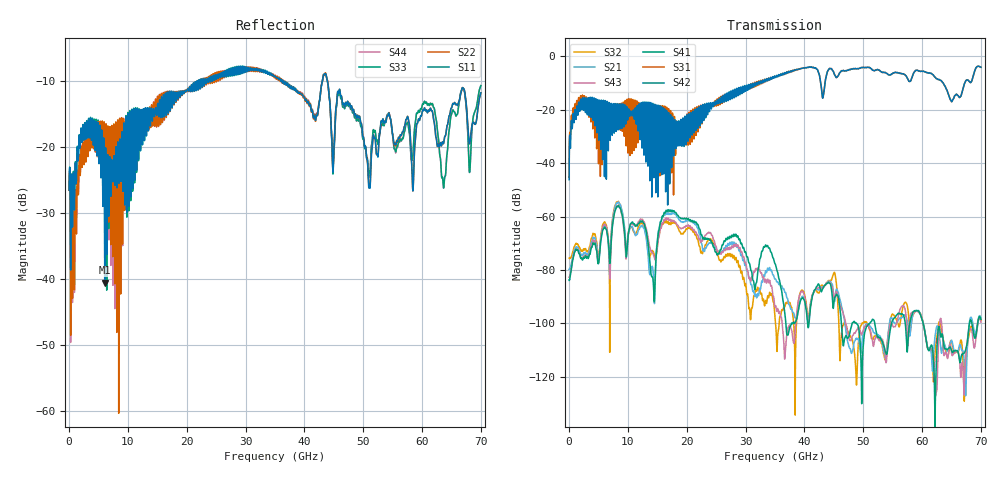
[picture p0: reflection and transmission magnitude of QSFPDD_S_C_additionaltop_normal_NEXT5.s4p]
! AWR Design Environment (8415) Thu Dec 20 13:45:36 2018
! Document = 'CHANNEL TEST'
! nPorts: 4, nXvals: 7001
# HZ S DB R 50
!Freq DBS11 AngS11 DBS12 AngS12 DBS13 AngS13 DBS14 AngS14
!	DBS21 AngS21 DBS22 AngS22 DBS23 AngS23 DBS24 AngS24
!	DBS31 AngS31 DBS32 AngS32 DBS33 AngS33 DBS34 AngS34
!	DBS41 AngS41 DBS42 AngS42 DBS43 AngS43 DBS44 AngS44
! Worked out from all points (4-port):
!   7000 points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, 10 MHz to 70 GHz, reference 50 ohm
!   strongest paths, dB at 10 MHz, 17.51 GHz, 35.01 GHz, 52.51 GHz, 70 GHz:
!     S42: -46.2, -26.2, -7.4, -5.0, -4.0
!     S31: -45.3, -23.9, -7.5, -5.0, -4.0
!     S41: -83.8, -57.6, -77.7, -105.1, -98.4
!     S43: -82.7, -61.3, -93.8, -105.6, -99.6
!     S21: -79.7, -58.6, -83.4, -104.3, -97.8
!     S32: -75.6, -62.1, -98.1, -105.1, -98.9
!   lowest |S11| = -40.5 dB at 6.06 GHz (marker M1), VSWR 1.02, Z = 49.4 + j0.738 ohm
!   |S11| at or under -10 dB: start of sweep to 21.77 GHz; 36.5 GHz to 43.04 GHz (6.538 GHz wide, 16.4 % of centre); 43.94 GHz to end of sweep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
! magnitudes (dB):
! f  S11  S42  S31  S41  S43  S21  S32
! 10 MHz  -26.5  -46.2  -45.3  -83.8  -82.7  -79.7  -75.6
! 1.64 GHz  -19.8  -17.2  -15.4  -73.6  -73.5  -72.6  -71.3
! 6.06 GHz  -40.5  -24.8  -18.8  -63.9  -62.8  -63.1  -62.0
! 13.94 GHz  -14.3  -17.9  -19.4  -81.6  -73.0  -79.4  -73.7
! 17.13 GHz  -13.3  -31.6  -29.2  -57.5  -60.9  -58.7  -62.2
! 31.21 GHz  -8.0  -10.1  -10.0  -83.4  -82.5  -87.8  -93.0
! 70 GHz  -11.8  -4.0  -4.0  -98.4  -99.6  -97.8  -98.9
